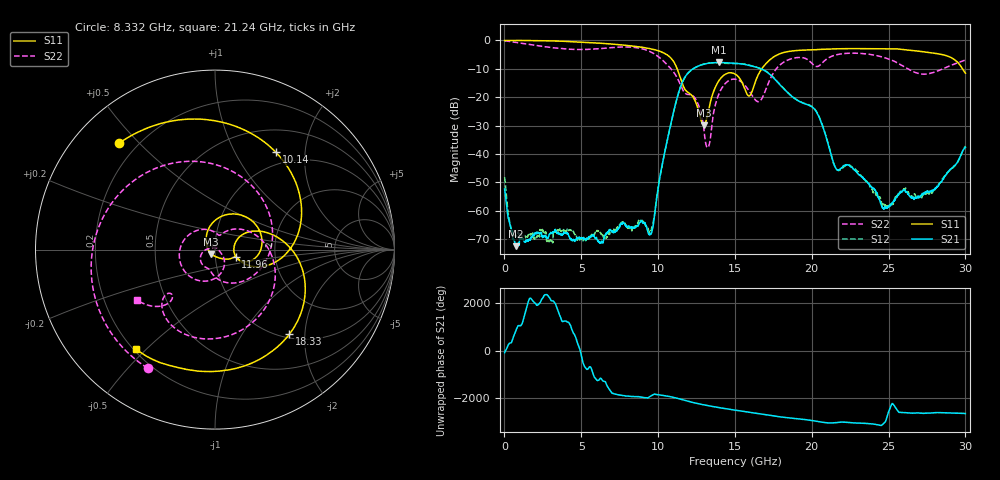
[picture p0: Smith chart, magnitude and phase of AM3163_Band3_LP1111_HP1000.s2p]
!Agilent Technologies,E8364B,MY43040894,A.07.50.67
!Agilent E8364B: A.07.50.67
!Date: Thursday, August 20, 2020 12:18:37
!Correction: S11(Full 2 Port(1,2))
!S21(Full 2 Port(1,2))
!S12(Full 2 Port(1,2))
!S22(Full 2 Port(1,2))
!S2P File: Measurements: S11, S21, S12, S22:
# Hz S  dB  R 50
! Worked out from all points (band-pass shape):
!   3201 points, 10 MHz to 30 GHz, reference 50 ohm
!   highest |S21| = -7.77 dB at 13.96 GHz (marker M1); lowest = -72.6 dB at 750.4 MHz (marker M2)
!   |S21| within 3 dB of the highest: 12.08 GHz to 16.98 GHz (4.899 GHz wide, 33.7 % of centre)
!   lowest |S11| = -29.9 dB at 12.96 GHz (marker M3), VSWR 1.07, Z = 47.9 - j2.33 ohm
!   |S11| at or under -10 dB: 11.24 GHz to 16.75 GHz (5.505 GHz wide, 39.3 % of centre); 29.8 GHz to end of sweep
!   |S22| runs from -37.8 to -0.1 dB; largest |S21 - S12| = 0.012
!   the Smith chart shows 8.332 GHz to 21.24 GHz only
!   S11 on the Smith chart (normalised r, x): 8.332 GHz: 0.13, +0.44; 10.14 GHz: 0.81, +1.48; 11.96 GHz: 1.25, -0.10; 18.33 GHz: 1.07, -1.67; 21.24 GHz: 0.21, -0.47
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1e7  -0.02 -1.9  -52.39 -87.8  -48.23 -33.3  -0.15 -4.9
7.503781e8  -0.01 -20.3  -72.55 129.4  -68.91 -142.0  -0.72 -51.4
2.755959e9  -0.11 -74.7  -69.75 -160.0  -70.75 170.6  -2.29 -168.1
5.014581e9  -0.58 -134.0  -69.52 126.1  -70.02 72.7  -3.20 72.8
6.617172e9  -1.12 -176.8  -68.03 55.6  -69.59 -57.5  -2.70 -16.7
8.332225e9  -1.96 131.9  -66.01 -131.6  -66.77 -132.7  -2.39 -119.5
9.513081e9  -2.94 87.8  -68.33 -115.3  -67.33 -156.4  -4.03 154.9
1.000979e10  -3.64 64.8  -51.79 -58.3  -51.85 -59.8  -5.71 108.8
1.0141e10  -3.88 58.0  -47.35 -71.0  -47.59 -71.9  -6.27 94.9
1.195914e10  -18.33 -19.1  -11.41 25.8  -11.48 26.2  -19.04 -113.4
1.296193e10  -29.88 -130.7  -8.38 -120.3  -8.36 -120.1  -30.35 168.1
1.328058e10  -24.60 143.9  -8.03 -160.0  -8.02 -160.1  -37.49 52.7
1.396472e10  -14.13 75.6  -7.77 121.8  -7.92 121.6  -18.78 -65.6
1.5005e10  -11.82 1.0  -8.05 16.0  -8.15 17.6  -13.65 -153.7
1.591407e10  -19.57 -0.1  -8.75 -72.9  -8.67 -72.2  -17.73 119.6
1.65701e10  -11.56 23.0  -9.74 -136.7  -9.73 -136.0  -21.57 72.7
1.833202e10  -4.04 -48.7  -17.87 63.0  -17.80 63.3  -7.18 -53.4
2.000958e10  -3.30 -99.6  -23.39 -62.0  -23.26 -61.7  -8.08 -136.9
2.12373e10  -2.99 -128.5  -39.93 -165.3  -39.69 -163.7  -5.72 -147.1
2.500479e10  -3.01 144.9  -58.64 -50.4  -58.16 -7.7  -6.56 68.2
2.740399e10  -4.10 77.9  -53.61 -114.4  -53.98 -107.4  -11.87 -88.2
3e10  -11.53 -28.2  -37.67 -127.5  -37.22 -125.7  -6.94 131.0
